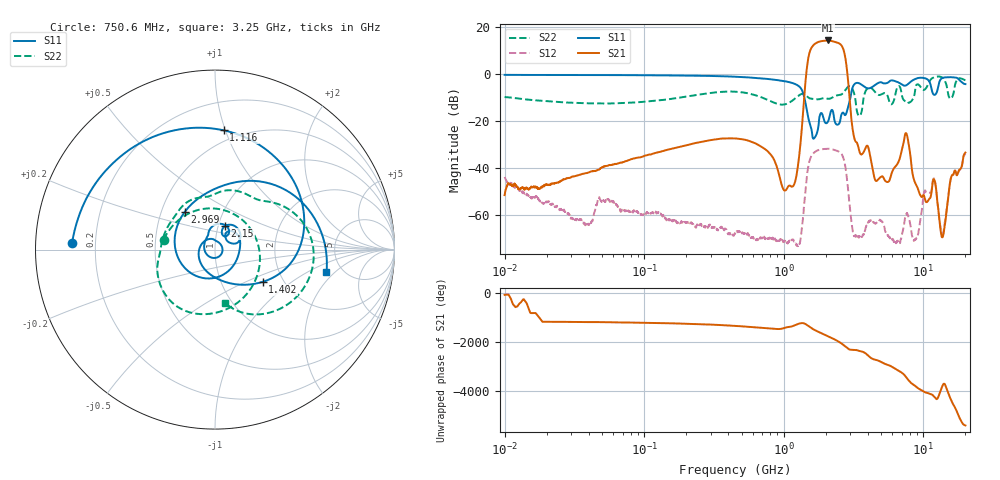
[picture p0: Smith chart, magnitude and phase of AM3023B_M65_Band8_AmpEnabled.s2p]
!Agilent Technologies,E8364B,MY43040894,A.07.50.67
!Agilent E8364B: A.07.50.67
!Date: Tuesday, October 27, 2020 10:54:11
!Correction: S11(Full 2 Port(1,2))
!S21(Full 2 Port(1,2))
!S12(Full 2 Port(1,2))
!S22(Full 2 Port(1,2))
!S2P File: Measurements: S11, S21, S12, S22:Log Frequency Sweep
# Hz S  dB  R 50
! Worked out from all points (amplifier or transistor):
!   3201 points, 10 MHz to 20 GHz, reference 50 ohm
!   highest |S21| = 14.4 dB at 2.065 GHz (marker M1)
!   |S21| within 3 dB of that: 1.584 GHz to 2.64 GHz (1.056 GHz wide, 50 % of centre)
!   unconditionally stable (mu >= 1): start of sweep to end of sweep
!   at 35.47 MHz: K = 6658.24, MAG = -31.5 dB, |S12| = -62.3 dB
!   at 447.2 MHz: K = 5244.26, MAG = -20.0 dB, |S12| = -67.9 dB
!   at 20 GHz: K = 332.07, MAG = -28.0 dB, |S12| = -34.0 dB
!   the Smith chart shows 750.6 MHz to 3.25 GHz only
!   S11 on the Smith chart (normalised r, x): 750.6 MHz: 0.11, +0.02; 1.116 GHz: 0.41, +0.99; 1.402 GHz: 1.57, -0.63; 2.15 GHz: 1.08, +0.29; 2.969 GHz: 0.66, +0.30; 3.25 GHz: 3.75, -1.59
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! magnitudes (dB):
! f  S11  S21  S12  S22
! 10 MHz  -0.3  -51.7  -43.9  -9.8
! 35.55 MHz  -0.4  -42.7  -62.6  -12.4
! 126.1 MHz  -0.5  -33.3  -58.9  -11.2
! 447.2 MHz  -1.1  -27.4  -67.9  -7.5
! 750.6 MHz  -2.0  -32.5  -70.3  -10.7
! 1.116 GHz  -3.5  -47.8  -71.0  -11.9
! 1.248 GHz  -4.6  -41.3  -73.4  -9.6
! 1.402 GHz  -9.9  -9.6  -55.1  -8.7
! 1.59 GHz  -24.6  11.6  -34.6  -10.5
! 2.065 GHz  -20.4  14.4  -31.9  -10.5
! 2.15 GHz  -16.9  14.3  -31.9  -10.4
! 2.662 GHz  -16.4  10.9  -35.5  -8.0
! 2.969 GHz  -11.4  -11.8  -56.5  -5.2
! 3.25 GHz  -4.0  -28.5  -69.3  -10.4
! 5.639 GHz  -3.4  -45.9  -69.4  -10.7
! 7.57 GHz  -4.7  -25.5  -60.0  -11.7
! 8.627 GHz  -2.2  -45.7  -71.0  -8.8
! 9.487 GHz  -1.5  -51.6  -62.7  -5.2
! 11.92 GHz  -8.8  -45.0  -44.5  -1.3
! 13.71 GHz  -1.6  -69.7  -68.4  -1.5
! 15.85 GHz  -1.3  -43.9  -44.0  -10.3
! 20 GHz  -4.2  -33.5  -34.0  -2.6
